|   National Semiconductor
|   DS90UH926QSQ
[IBIS Ver]   4.1
[File name]   ds90uh926qsq.ibs
[File Rev]   1.0
[Date]   02/03/2011
[Source]   SPICE to IBIS Translation
[Notes]
CML Inputs are NOT SUPPORTED in this version of the IBIS model
The following IBIS Parser notes and warnings have been reviewed and are
considered very minor and should not cause any modeling issues:
WARNING (line 6359) - GND Clamp Minimum data is non-monotonic
WARNING (line 6362) - GND Clamp Typical data is non-monotonic
WARNING (line 6365) - GND Clamp Maximum data is non-monotonic
WARNING (line 6504) - POWER Clamp Minimum data is non-monotonic
WARNING (line 6513) - POWER Clamp Typical data is non-monotonic
WARNING (line 6513) - POWER Clamp Maximum data is non-monotonic
WARNING (line 10818) - GND Clamp Minimum data is non-monotonic
WARNING (line 10819) - GND Clamp Typical data is non-monotonic
WARNING (line 10819) - GND Clamp Maximum data is non-monotonic
WARNING (line 10964) - POWER Clamp Minimum data is non-monotonic
WARNING (line 10969) - POWER Clamp Typical data is non-monotonic
WARNING (line 10969) - POWER Clamp Maximum data is non-monotonic
WARNING (line 15272) - GND Clamp Minimum data is non-monotonic
WARNING (line 15273) - GND Clamp Typical data is non-monotonic
WARNING (line 15274) - GND Clamp Maximum data is non-monotonic
WARNING (line 15418) - POWER Clamp Minimum data is non-monotonic
WARNING (line 15422) - POWER Clamp Maximum data is non-monotonic
WARNING (line 15423) - POWER Clamp Typical data is non-monotonic
WARNING (line 19726) - GND Clamp Minimum data is non-monotonic
WARNING (line 19727) - GND Clamp Typical data is non-monotonic
WARNING (line 19727) - GND Clamp Maximum data is non-monotonic
WARNING (line 19872) - POWER Clamp Minimum data is non-monotonic
WARNING (line 19877) - POWER Clamp Typical data is non-monotonic
WARNING (line 19877) - POWER Clamp Maximum data is non-monotonic
WARNING (line 24228) - GND Clamp Minimum data is non-monotonic
WARNING -
   Model LVCMOS_DATA_IN_33V: POWER Clamp : Maximum value never becomes zero
WARNING (line 24446) - GND Clamp Minimum data is non-monotonic
WARNING -
   Model LVCMOS_PWDN_3325V_33V: POWER Clamp : Typical value never becomes zero
WARNING -
   Model LVCMOS_PWDN_3325V_33V: POWER Clamp : Minimum value never becomes zero
WARNING -
   Model LVCMOS_PWDN_3325V_33V: POWER Clamp : Maximum value never becomes zero
WARNING (line 24664) - GND Clamp Minimum data is non-monotonic
WARNING -
   Model LVCMOS_PWDN_I_33V: POWER Clamp : Typical value never becomes zero
WARNING -
   Model LVCMOS_PWDN_I_33V: POWER Clamp : Minimum value never becomes zero
WARNING -
   Model LVCMOS_PWDN_I_33V: POWER Clamp : Maximum value never becomes zero
WARNING (line 24828) - GND Clamp Maximum data is non-monotonic
WARNING (line 24830) - GND Clamp Typical data is non-monotonic
WARNING (line 24835) - GND Clamp Minimum data is non-monotonic
WARNING (line 24977) - POWER Clamp Typical data is non-monotonic
WARNING (line 24979) - POWER Clamp Maximum data is non-monotonic
WARNING (line 24980) - POWER Clamp Minimum data is non-monotonic
WARNING (line 29287) - GND Clamp Maximum data is non-monotonic
WARNING (line 29289) - GND Clamp Typical data is non-monotonic
WARNING (line 29293) - GND Clamp Minimum data is non-monotonic
WARNING (line 29438) - POWER Clamp Maximum data is non-monotonic
WARNING (line 29439) - POWER Clamp Minimum data is non-monotonic
WARNING (line 29441) - POWER Clamp Typical data is non-monotonic
WARNING (line 33741) - GND Clamp Maximum data is non-monotonic
WARNING (line 33743) - GND Clamp Typical data is non-monotonic
WARNING (line 33747) - GND Clamp Minimum data is non-monotonic
WARNING (line 33892) - POWER Clamp Maximum data is non-monotonic
WARNING (line 33893) - POWER Clamp Minimum data is non-monotonic
WARNING (line 33895) - POWER Clamp Typical data is non-monotonic
WARNING (line 38249) - GND Clamp Minimum data is non-monotonic
WARNING (line 38412) - GND Clamp Maximum data is non-monotonic
WARNING (line 38415) - GND Clamp Typical data is non-monotonic
WARNING (line 38420) - GND Clamp Minimum data is non-monotonic
WARNING (line 38558) - POWER Clamp Maximum data is non-monotonic
WARNING (line 38562) - POWER Clamp Typical data is non-monotonic
WARNING (line 38565) - POWER Clamp Minimum data is non-monotonic
WARNING (line 42921) - GND Clamp Minimum data is non-monotonic
WARNING -
   Model LVCMOS_PWDN_3325V_18V: POWER Clamp : Typical value never becomes zero
WARNING -
   Model LVCMOS_PWDN_3325V_18V: POWER Clamp : Maximum value never becomes zero
WARNING (line 43139) - GND Clamp Minimum data is non-monotonic
WARNING -
   Combined Pullup for Model: LVCMOS_DATA_2_18V Typical data is non-monotonic
WARNING - Combined Pulldown for Model: LVCMOS_DATA_2_18V Minimum data is non-monotonic
WARNING -
   Combined Pullup for Model: LVCMOS_DATA_2_18V Minimum data is non-monotonic
WARNING - Model LVCMOS_DATA_2_18V: The [Rising Waveform]
   with [R_fixture]=500 Ohms and [V_fixture_min]=0V
   has MIN column DC endpoints of  0.00V and  1.49v, but
   an equivalent load applied to the model's I-V tables yields
   different voltages ( 0.04V and  1.50V),
   a difference of  3.05% and  0.95%, respectively.
WARNING - Model LVCMOS_DATA_2_18V: The [Rising Waveform]
   with [R_fixture]=500 Ohms and [V_fixture_min]=1.62V
   has MIN column DC endpoints of  0.12V and  1.62v, but
   an equivalent load applied to the model's I-V tables yields
   different voltages ( 0.17V and  1.62V),
   a difference of  2.95% and  0.01%, respectively.
WARNING - Model LVCMOS_DATA_2_18V: The [Falling Waveform]
   with [R_fixture]=500 Ohms and [V_fixture_min]=0V
   has MIN column DC endpoints of  0.00V and  1.49v, but
   an equivalent load applied to the model's I-V tables yields
   different voltages ( 0.04V and  1.50V),
   a difference of  3.05% and  0.27%, respectively.
WARNING - Model LVCMOS_DATA_2_18V: The [Falling Waveform]
   with [R_fixture]=500 Ohms and [V_fixture_min]=1.62V
   has MIN column DC endpoints of  0.12V and  1.62v, but
   an equivalent load applied to the model's I-V tables yields
   different voltages ( 0.17V and  1.62V),
   a difference of  2.95% and  0.01%, respectively.
WARNING - Combined Pulldown for Model: LVCMOS_DATA_2_18V Maximum data is non-monotonic
WARNING -
   Combined Pullup for Model: LVCMOS_DATA_2_18V Maximum data is non-monotonic
WARNING - Combined Pulldown for Model: LVCMOS_DATA_1_18V Typical data is non-monotonic
WARNING -
   Combined Pullup for Model: LVCMOS_DATA_1_18V Typical data is non-monotonic
WARNING - Combined Pulldown for Model: LVCMOS_DATA_1_18V Minimum data is non-monotonic
WARNING - Model LVCMOS_DATA_1_18V: The [Rising Waveform]
   with [R_fixture]=500 Ohms and [V_fixture_min]=0V
   has MIN column DC endpoints of  0.00V and  1.48v, but
   an equivalent load applied to the model's I-V tables yields
   different voltages ( 0.04V and  1.50V),
   a difference of  2.62% and  0.97%, respectively.
WARNING - Model LVCMOS_DATA_1_18V: The [Rising Waveform]
   with [R_fixture]=500 Ohms and [V_fixture_min]=1.62V
   has MIN column DC endpoints of  0.12V and  1.62v, but
   an equivalent load applied to the model's I-V tables yields
   different voltages ( 0.16V and  1.62V),
   a difference of  2.53% and  0.04%, respectively.
WARNING - Model LVCMOS_DATA_1_18V: The [Falling Waveform]
   with [R_fixture]=500 Ohms and [V_fixture_min]=0V
   has MIN column DC endpoints of  0.00V and  1.49v, but
   an equivalent load applied to the model's I-V tables yields
   different voltages ( 0.04V and  1.50V),
   a difference of  2.61% and  0.24%, respectively.
WARNING - Model LVCMOS_DATA_1_18V: The [Falling Waveform]
   with [R_fixture]=500 Ohms and [V_fixture_min]=1.62V
   has MIN column DC endpoints of  0.12V and  1.62v, but
   an equivalent load applied to the model's I-V tables yields
   different voltages ( 0.16V and  1.62V),
   a difference of  2.52% and  0.04%, respectively.
WARNING -
   Combined Pullup for Model: LVCMOS_DATA_1_18V Maximum data is non-monotonic
WARNING -
   Combined Pullup for Model: LVCMOS_DATA_18V Typical data is non-monotonic
WARNING -
   Combined Pulldown for Model: LVCMOS_DATA_18V Minimum data is non-monotonic
WARNING -
   Combined Pullup for Model: LVCMOS_DATA_18V Minimum data is non-monotonic
WARNING - Model LVCMOS_DATA_18V: The [Rising Waveform]
   with [R_fixture]=500 Ohms and [V_fixture_min]=0V
   has MIN column DC endpoints of  0.00V and  1.48v, but
   an equivalent load applied to the model's I-V tables yields
   different voltages ( 0.04V and  1.50V),
   a difference of  2.60% and  0.96%, respectively.
WARNING - Model LVCMOS_DATA_18V: The [Rising Waveform]
   with [R_fixture]=500 Ohms and [V_fixture_min]=1.62V
   has MIN column DC endpoints of  0.12V and  1.62v, but
   an equivalent load applied to the model's I-V tables yields
   different voltages ( 0.16V and  1.62V),
   a difference of  2.51% and  0.05%, respectively.
WARNING - Model LVCMOS_DATA_18V: The [Falling Waveform]
   with [R_fixture]=500 Ohms and [V_fixture_min]=0V
   has MIN column DC endpoints of  0.00V and  1.49v, but
   an equivalent load applied to the model's I-V tables yields
   different voltages ( 0.04V and  1.50V),
   a difference of  2.59% and  0.23%, respectively.
WARNING - Model LVCMOS_DATA_18V: The [Falling Waveform]
   with [R_fixture]=500 Ohms and [V_fixture_min]=1.62V
   has MIN column DC endpoints of  0.12V and  1.62v, but
   an equivalent load applied to the model's I-V tables yields
   different voltages ( 0.16V and  1.62V),
   a difference of  2.51% and  0.05%, respectively.
WARNING -
   Combined Pullup for Model: LVCMOS_DATA_18V Maximum data is non-monotonic
WARNING -
   Combined Pulldown for Model: LVCMOS_CLK_18V Typical data is non-monotonic
WARNING -
   Combined Pullup for Model: LVCMOS_CLK_18V Typical data is non-monotonic
WARNING -
   Combined Pulldown for Model: LVCMOS_CLK_18V Minimum data is non-monotonic
WARNING -
   Combined Pullup for Model: LVCMOS_CLK_18V Minimum data is non-monotonic
WARNING -
   Combined Pulldown for Model: LVCMOS_CLK_18V Maximum data is non-monotonic
WARNING -
   Combined Pullup for Model: LVCMOS_CLK_18V Maximum data is non-monotonic
WARNING - Model LVCMOS_CLK_18V: The [Rising Waveform]
   with [R_fixture]=500 Ohms and [V_fixture_max]=1.98V
   has MAX column DC endpoints of  0.08V and  1.98v, but
   an equivalent load applied to the model's I-V tables yields
   different voltages ( 0.08V and  1.93V),
   a difference of  0.07% and  2.60%, respectively.
WARNING - Combined Pulldown for Model: LVCMOS_DATA_2_33V Typical data is non-monotonic
WARNING -
   Combined Pullup for Model: LVCMOS_DATA_2_33V Typical data is non-monotonic
WARNING - Combined Pulldown for Model: LVCMOS_DATA_2_33V Minimum data is non-monotonic
WARNING -
   Combined Pullup for Model: LVCMOS_DATA_2_33V Minimum data is non-monotonic
WARNING - Combined Pulldown for Model: LVCMOS_DATA_2_33V Maximum data is non-monotonic
WARNING - Model LVCMOS_DATA_2_33V: The [Rising Waveform]
   with [R_fixture]=500 Ohms and [V_fixture_max]=0V
   has MAX column DC endpoints of  0.00V and  3.48v, but
   an equivalent load applied to the model's I-V tables yields
   different voltages ( 0.08V and  3.48V),
   a difference of  2.31% and  0.19%, respectively.
WARNING - Model LVCMOS_DATA_2_33V: The [Rising Waveform]
   with [R_fixture]=500 Ohms and [V_fixture_max]=3.63V
   has MAX column DC endpoints of  0.14V and  3.63v, but
   an equivalent load applied to the model's I-V tables yields
   different voltages ( 0.22V and  3.63V),
   a difference of  2.27% and  0.00%, respectively.
WARNING - Model LVCMOS_DATA_2_33V: The [Falling Waveform]
   with [R_fixture]=500 Ohms and [V_fixture_max]=0V
   has MAX column DC endpoints of  0.00V and  3.48v, but
   an equivalent load applied to the model's I-V tables yields
   different voltages ( 0.08V and  3.48V),
   a difference of  2.31% and  0.13%, respectively.
WARNING - Model LVCMOS_DATA_2_33V: The [Falling Waveform]
   with [R_fixture]=500 Ohms and [V_fixture_max]=3.63V
   has MAX column DC endpoints of  0.14V and  3.63v, but
   an equivalent load applied to the model's I-V tables yields
   different voltages ( 0.22V and  3.63V),
   a difference of  2.24% and  0.00%, respectively.
WARNING - Combined Pulldown for Model: LVCMOS_DATA_1_33V Typical data is non-monotonic
WARNING -
   Combined Pullup for Model: LVCMOS_DATA_1_33V Typical data is non-monotonic
WARNING - Combined Pulldown for Model: LVCMOS_DATA_1_33V Minimum data is non-monotonic
WARNING -
   Combined Pullup for Model: LVCMOS_DATA_1_33V Minimum data is non-monotonic
WARNING -
   Combined Pulldown for Model: LVCMOS_DATA_33V Typical data is non-monotonic
WARNING -
   Combined Pullup for Model: LVCMOS_DATA_33V Typical data is non-monotonic
WARNING -
   Combined Pulldown for Model: LVCMOS_DATA_33V Minimum data is non-monotonic
WARNING -
   Combined Pullup for Model: LVCMOS_DATA_33V Minimum data is non-monotonic
WARNING - Model LVCMOS_DATA_33V: The [Rising Waveform]
   with [R_fixture]=500 Ohms and [V_fixture_max]=0V
   has MAX column DC endpoints of  0.00V and  3.48v, but
   an equivalent load applied to the model's I-V tables yields
   different voltages ( 0.07V and  3.48V),
   a difference of  2.14% and  0.15%, respectively.
WARNING - Model LVCMOS_DATA_33V: The [Rising Waveform]
   with [R_fixture]=500 Ohms and [V_fixture_max]=3.63V
   has MAX column DC endpoints of  0.14V and  3.63v, but
   an equivalent load applied to the model's I-V tables yields
   different voltages ( 0.22V and  3.63V),
   a difference of  2.11% and  0.06%, respectively.
WARNING - Model LVCMOS_DATA_33V: The [Falling Waveform]
   with [R_fixture]=500 Ohms and [V_fixture_max]=0V
   has MAX column DC endpoints of  0.00V and  3.48v, but
   an equivalent load applied to the model's I-V tables yields
   different voltages ( 0.07V and  3.48V),
   a difference of  2.14% and  0.08%, respectively.
WARNING - Model LVCMOS_DATA_33V: The [Falling Waveform]
   with [R_fixture]=500 Ohms and [V_fixture_max]=3.63V
   has MAX column DC endpoints of  0.14V and  3.63v, but
   an equivalent load applied to the model's I-V tables yields
   different voltages ( 0.22V and  3.63V),
   a difference of  2.08% and  0.06%, respectively.
WARNING -
   Combined Pulldown for Model: LVCMOS_CLK_33V Typical data is non-monotonic
WARNING -
   Combined Pullup for Model: LVCMOS_CLK_33V Typical data is non-monotonic
WARNING -
   Combined Pulldown for Model: LVCMOS_CLK_33V Minimum data is non-monotonic
WARNING -
   Combined Pullup for Model: LVCMOS_CLK_33V Minimum data is non-monotonic
WARNING -
   Combined Pulldown for Model: LVCMOS_CLK_33V Maximum data is non-monotonic
Errors  : 0
Warnings: 121
File Passed
[Disclaimer]
(C) Copyright National Semiconductor Corporation 2011
   All rights reserved
National Semiconductor Corporation hereby grants the
user of this IBIS model a non-exclusive, nontransferable
license to use this IBIS model under the following terms.
Before using this IBIS model, the user should read this
license.  If the user does not accept these terms,  the
IBIS model should be returned to National within 30 days.
The user is granted this license only to use the
IBIS model and is not granted rights to sell, load, rent,
lease or license the IBIS model in whole or in part, or in
modified form to anyone other than user. User may modify
the IBIS model to suit its specific applications but rights
to derivative works and such modifications shall belong to
National.
This IBIS model is provided on an "AS IS" basis and
National makes absolutely no warranty with respect to the
information contained herein.NATIONAL DISCLAIMS AND CUSTOMER
WAIVES ALL WARRANTIES, EXPRESS OR IMPLIED, INCLUDING
WARRANTIES OF MERCHANTABILITY OR FITNESS FOR A PARTICULAR
PURPOSE. The entire risk as to quality and performance is
with the Customer. ACCORDINGLY, IN NO EVENT SHALL THE
COMPANY BE LIABLE FOR ANY DAMAGES, WHETHER IN CONTRACT OR
TORT,INCLUDING ANY LOST PROFITS OR OTHER INCIDENTAL,
CONSEQUENTIAL, EXEMPLARY, OR PUNITIVE DAMAGES ARISING OUT
OF THE USE OR APPLICATION OF THE IBIS model provided in
this package.Further, National reserves the right to make
changes without notice to any product herein to improve
reliability, function, or design. National does not convey
any license under patent rights or any other intellectual
property rights, including those of third parties.
National is not obligated to provide maintenance or support
for the licensed IBIS model.
[Copyright]   Copyright 2011, National Semiconductor, All Rights Reserved
[Component]   DS90UH926QSQ
Si_location   Pin
Timing_location   Pin
[Manufacturer]   National Semiconductor
[Package]
R_pkg   0m   0m   0m
L_pkg   0n   0n   0n
C_pkg   0p   0p   0p
[PIN]   signal_name   model_name   R_pin   L_pin   C_pin
1   I2S_CLK   LVCMOS_CLK
2   SDA   NC
3   SCL   NC
4   CAPL12   NC
5   PCLK   LVCMOS_CLK
6   DE   LVCMOS_DATA
7   VS   LVCMOS_DATA
8   HS   LVCMOS_DATA_2
9   B7   LVCMOS_DATA
10   B6   LVCMOS_DATA
11   B5   LVCMOS_DATA
12   B4   LVCMOS_DATA
13   VDDIO   POWER
14   B3   LVCMOS_DATA
15   MODE_SEL   NC
16   BISTC   LVCMOS_DATA_IN
17   B2   LVCMOS_DATA
18   B1   LVCMOS_DATA_1
19   B0   LVCMOS_DATA_1
20   G7   LVCMOS_DATA
21   G6   LVCMOS_DATA
22   G5   LVCMOS_DATA
23   G4   LVCMOS_DATA
24   VDDIO   POWER
25   G3   LVCMOS_DATA
26   G2   LVCMOS_DATA
27   G1   LVCMOS_DATA
28   G0   LVCMOS_DATA
29   VDD33_B   POWER
30   I2S_WC   LVCMOS_DATA
31   OEN   LVCMOS_DATA_IN
32   LOCK   LVCMOS_DATA
33   R7   LVCMOS_DATA
34   R6   LVCMOS_DATA
35   R5   LVCMOS_DATA
36   R4   LVCMOS_DATA
37   R3   LVCMOS_DATA
38   VDDIO   POWER
39   R2   LVCMOS_DATA
40   R1   LVCMOS_DATA
41   R0   LVCMOS_DATA
42   PASS   LVCMOS_DATA
43   RES1   NC
44   BISTEN   LVCMOS_PWDN_3325V
45   I2S_DA   LVCMOS_DATA_2
46   OSS_SEL   LVCMOS_DATA_IN
47   RES0   NC
48   VDD33_A   POWER
49   RINp   NC
50   RINn   NC
51   CMF   NC
52   CMLOUTp   NC
53   CMLOUTn   NC
54   NC   NC
55   CAPR12   NC
56   IDx   NC
57   CAPP12   NC
58   CAPI2S   NC
59   PDB   LVCMOS_PWDN_I
60   MCLK   LVCMOS_CLK
DAP   GND   GND
|   Model Selectors
[Model Selector]  LVCMOS_CLK
LVCMOS_CLK_33V   3.3V output
LVCMOS_CLK_18V   1.8V output
[Model Selector]  LVCMOS_DATA
LVCMOS_DATA_33V   3.3V output
LVCMOS_DATA_18V   1.8V output
[Model Selector]  LVCMOS_DATA_1
LVCMOS_DATA_1_33V   3.3V output
LVCMOS_DATA_1_18V   1.8V output
[Model Selector]  LVCMOS_DATA_IN
LVCMOS_DATA_IN_33V   3.3V input
LVCMOS_DATA_IN_18V   1.8V input
[Model Selector]  LVCMOS_DATA_2
LVCMOS_DATA_2_33V   3.3V output
LVCMOS_DATA_2_18V   1.8V output
[Model Selector]  LVCMOS_PWDN_3325V
LVCMOS_PWDN_3325V_33V   3.3V input
LVCMOS_PWDN_3325V_18V   1.8V input
[Model Selector]  LVCMOS_PWDN_I
LVCMOS_PWDN_I_33V   3.3V input
LVCMOS_PWDN_I_18V   1.8V input
[Define Package Model]  llp60_v2_DS90UH926QSQ
[Manufacturer]  Unknown
[OEM]  Unknown
[Description]   Ansoft Q3D Extractor Pkg Model - Buildsheet# DS90UH926QSQ
[Number Of Pins]  60
[Pin Numbers]
61   | 61 = DAP
1   | 1 = L1
2   | 2 = L2
3   | 3 = L3
4   | 4 = L4
5   | 5 = L5
6   | 6 = L6
7   | 7 = L7
8   | 8 = L8
9   | 9 = L9
10   | 10 = L10
11   | 11 = L11
12   | 12 = L12
13   | 13 = L13
14   | 14 = L14
15   | 15 = L15
16   | 16 = L16
17   | 17 = L17
18   | 18 = L18
19   | 19 = L19
20   | 20 = L20
21   | 21 = L21
22   | 22 = L22
23   | 23 = L23
24   | 24 = L24
25   | 25 = L25
26   | 26 = L26
27   | 27 = L27
28   | 28 = L28
29   | 29 = L29
30   | 30 = L30
31   | 31 = L31
32   | 32 = L32
33   | 33 = L33
34   | 34 = L34
35   | 35 = L35
36   | 36 = L36
37   | 37 = L37
38   | 38 = L38
39   | 39 = L39
40   | 40 = L40
41   | 41 = L41
42   | 42 = L42
43   | 43 = L43
44   | 44 = L44
45   | 45 = L45
46   | 46 = L46
47   | 47 = L47
48   | 48 = L48
49   | 49 = L49
50   | 50 = L50
51   | 51 = L51
52   | 52 = L52
53   | 53 = L53
55   | 55 = L55
56   | 56 = L56
57   | 57 = L57
58   | 58 = L58
59   | 59 = L59
60   | 60 = L60
[Model Data]
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[End Model Data]
[End Package Model]
| Models and submodels in the file (14): LVCMOS_CLK_33V (3-state), LVCMOS_DATA_33V (3-state), LVCMOS_DATA_1_33V (3-state), LVCMOS_DATA_2_33V (3-state), LVCMOS_DATA_IN_33V (Input), LVCMOS_PWDN_3325V_33V (Input), LVCMOS_PWDN_I_33V (Input), LVCMOS_CLK_18V (3-state), LVCMOS_DATA_18V (3-state), LVCMOS_DATA_1_18V (3-state), LVCMOS_DATA_IN_18V (Input), LVCMOS_DATA_2_18V (3-state), LVCMOS_PWDN_3325V_18V (Input), LVCMOS_PWDN_I_18V (Input)
